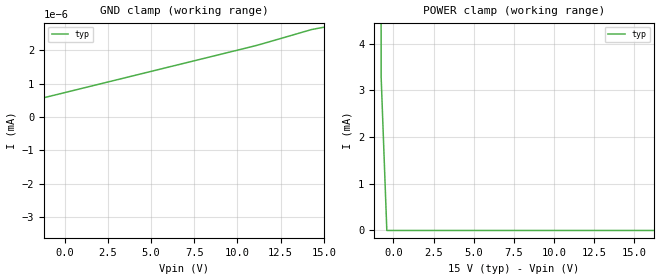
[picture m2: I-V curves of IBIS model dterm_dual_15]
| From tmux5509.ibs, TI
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| dterm_dual_15
[Model]   dterm_dual_15
Model_type   Terminator
|   typ   min   max
C_comp   6.362683e-12   NA   NA
[Voltage Range]   15   NA   NA
[Temperature Range]   27   NA   NA
[Power Clamp Reference]   15   NA   NA
[GND Clamp Reference]   0   NA   NA
[GND Clamp]
|   Voltage   I(typ)   I(min)   I(max)
-20V      -2.839A    NA         NA
-15.4V    -221.5nA   NA         NA
-15.05V   -1.213nA   NA         NA
-14.34V   -1.14nA    NA         NA
-11.16V   -686pA     NA         NA
11.11V    2.144nA    NA         NA
14.29V    2.618nA    NA         NA
15V       2.688nA    NA         NA
[POWER Clamp]
|   Voltage   I(typ)   I(min)   I(max)
-5V       7.432A     NA         NA
-1.111V   237.2mA    NA         NA
-757.6mV  3.292mA    NA         NA
-404mV    146.4nA    NA         NA
30V       -2.267nA   NA         NA
